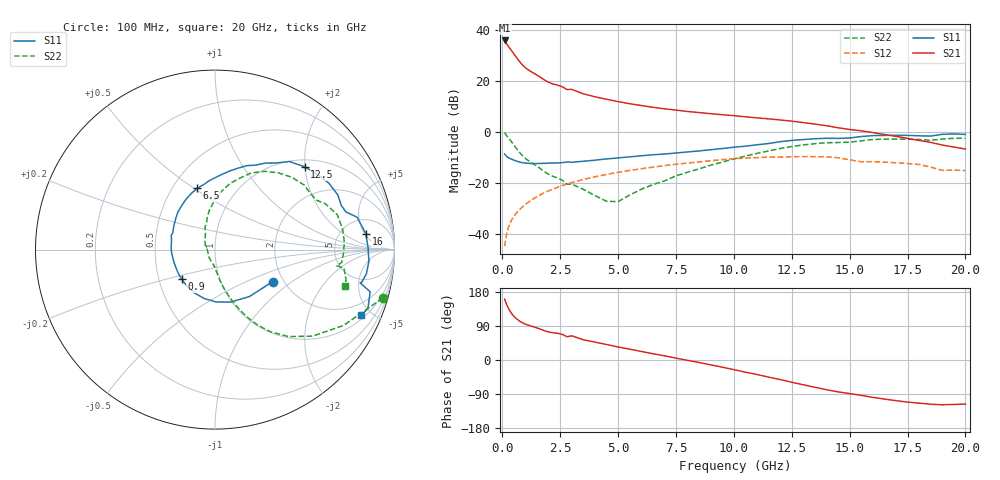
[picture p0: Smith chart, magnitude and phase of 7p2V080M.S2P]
! Infineon Technologies  Discrete & RF Semiconductors
! bfp620
! VCE =  2.0 V,  IC =  80 mA
! Common Emitter S-Parameters:  Sep 2002
# GHz  S  MA  R  50
!  f  S11  S21  S12  S22
! GHz  MAG  ANG  MAG  ANG  MAG  ANG  MAG  ANG
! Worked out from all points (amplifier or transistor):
!   59 points, 100 MHz to 20 GHz, reference 50 ohm
!   highest |S21| = 35.9 dB at 100 MHz (marker M1)
!   |S21| within 3 dB of that: start of sweep to 318.2 MHz
!   unconditionally stable (mu >= 1): 1.964 GHz to 2.361 GHz; 2.48 GHz to 9.902 GHz; 17.16 GHz to end of sweep
!   at 1 GHz: K = 0.89, MSG = 26.8 dB, |S12| = -28.5 dB
!   at 5.5 GHz: K = 1.04, MAG = 11.9 dB, |S12| = -15.1 dB
!   at 20 GHz: K = 1.26, MAG = 1.2 dB, |S12| = -15.2 dB
!   S11 on the Smith chart (normalised r, x): 100 MHz: 1.75, -0.72; 900 MHz: 0.65, -0.23; 6.5 GHz: 0.66, +0.52; 12.5 GHz: 1.16, +1.99; 16 GHz: 9, +5; 20 GHz: 1.20, -4.35
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0.1  0.3672 -29.1  62.52 160.5  0.0057 80.7  0.9728 -16.1
0.2  0.3244 -53.7  52.52 144.7  0.0107 74.9  0.8312 -30.6
0.3  0.3052 -73.4  45.41 132.4  0.0149 72.4  0.7263 -41.6
0.4  0.2914 -89.2  39.44 122.9  0.0186 70.8  0.6355 -49.7
0.5  0.279 -102.4  34.13 115.5  0.0219 69.8  0.5537 -55.9
0.6  0.2681 -113.7  29.49 109.5  0.0252 69.0  0.4816 -60.6
0.7  0.2594 -123.5  25.6 104.7  0.0283 68.4  0.4206 -64.3
0.9  0.248 -138.8  20.06 97.3  0.0346 67.5  0.3321 -69.5
1.2  0.2402 -154.0  15.71 90.4  0.0441 66.1  0.2592 -74.1
2  0.2439 179.0  9.412 74.0  0.0695 60.8  0.1469 -83.4
2.8  0.2565 161.9  6.781 61.3  0.0947 54.0  0.0933 -92.3
3  0.2534 158.3  6.859 63.9  0.101 52.1  0.0946 -91.4
3.5  0.2652 149.7  5.599 53.5  0.1164 47.4  0.0743 -102.9
5  0.3083 126.7  3.937 34.4  0.1608 32.9  0.0427 -177.1
6.5  0.3557 106.1  3.045 16.6  0.2028 18.2  0.092 126.0
7  0.3675 99.9  2.842 11.1  0.2171 13.4  0.1088 118.9
10.5  0.524 64.0  1.982 -32.2  0.3058 -26.3  0.3338 82.7
12.5  0.6803 42.7  1.626 -58.7  0.3265 -49.9  0.5176 57.4
13.5  0.7346 30.2  1.425 -71.9  0.3263 -62.7  0.5877 43.3
16  0.8452 6.0  0.972 -98.6  0.2602 -86.6  0.7088 15.9
17  0.8598 -4.4  0.82 -107.3  0.2476 -94.6  0.7216 3.6
20  0.8934 -24.2  0.461 -116.2  0.1737 -104.2  0.7527 -15.8
